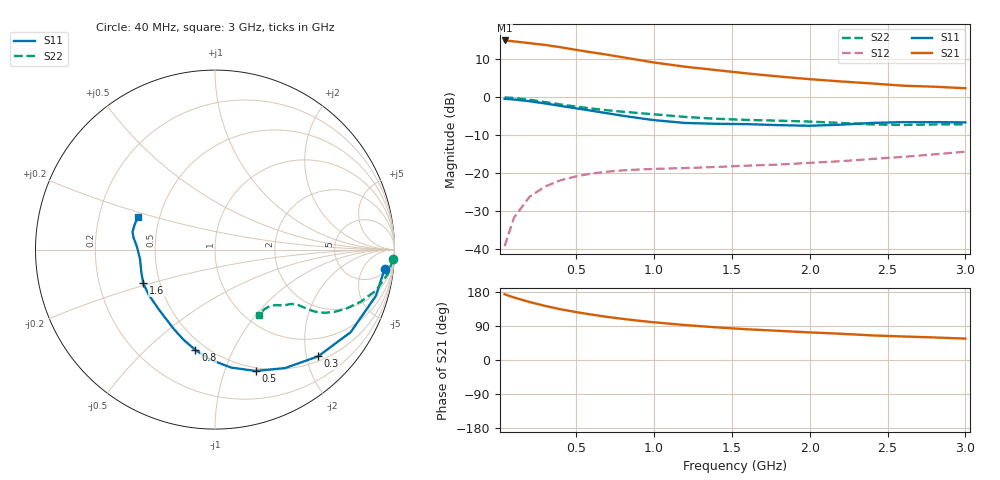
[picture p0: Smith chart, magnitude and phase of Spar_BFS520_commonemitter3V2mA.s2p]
! Filename:  BFS520A.S2P  Version:  4.0
! NXP part #: BFS520  Date: Jun 1994
! Bias condition: Vce=3V, Ic=2mA
#  MHz  S  MA  R  50
! Freq  S11  S21  S12  S22  !GUM [dB]
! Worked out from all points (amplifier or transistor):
!   21 points, 40 MHz to 3 GHz, reference 50 ohm
!   highest |S21| = 14.9 dB at 40 MHz (marker M1)
!   |S21| within 3 dB of that: start of sweep to 580.8 MHz
!   unconditionally stable (mu >= 1): 1.322 GHz to end of sweep
!   at 300 MHz: K = 0.28, MSG = 18.6 dB, |S12| = -23.5 dB
!   at 1 GHz: K = 0.78, MSG = 14.0 dB, |S12| = -18.9 dB
!   at 3 GHz: K = 1.19, MAG = 5.7 dB, |S12| = -14.3 dB
!   S11 on the Smith chart (normalised r, x): 40 MHz: 7, -15; 300 MHz: 0.59, -2.22; 500 MHz: 0.47, -1.28; 800 MHz: 0.44, -0.73; 1.6 GHz: 0.40, -0.19; 3 GHz: 0.38, +0.18
40  0.951 -6.5  5.567 173.5  0.011 85.2  0.992 -3.1
100  0.933 -16.0  5.416 165.0  0.026 79.0  0.976 -7.6
200  0.885 -31.3  5.128 153.0  0.049 69.6  0.925 -14.3
300  0.827 -46.0  4.862 142.8  0.067 62.0  0.862 -19.7
400  0.767 -59.4  4.532 133.8  0.081 56.2  0.803 -24.1
500  0.713 -71.5  4.186 126.4  0.091 51.9  0.751 -27.5
600  0.663 -82.3  3.885 119.8  0.099 48.9  0.708 -29.8
700  0.614 -92.3  3.615 113.7  0.105 47.1  0.673 -31.3
800  0.57 -101.0  3.342 108.5  0.109 45.9  0.644 -32.1
900  0.532 -109.2  3.088 103.7  0.112 44.9  0.619 -32.6
1000  0.499 -117.3  2.857 99.5  0.114 44.7  0.595 -33.0
1200  0.458 -132.8  2.514 92.2  0.117 45.2  0.55 -33.8
1400  0.447 -145.5  2.27 86.2  0.121 47.0  0.52 -35.6
1600  0.442 -154.8  2.05 81.0  0.126 49.3  0.502 -37.9
1800  0.429 -163.2  1.871 77.0  0.13 52.8  0.491 -39.4
2000  0.421 -172.9  1.725 72.8  0.137 56.2  0.478 -40.5
2200  0.435 178.0  1.61 69.3  0.144 59.9  0.458 -42.4
2400  0.459 171.6  1.514 64.9  0.154 62.9  0.438 -46.1
2600  0.47 167.8  1.416 62.1  0.164 65.4  0.431 -50.9
2800  0.469 163.3  1.373 59.5  0.177 68.6  0.438 -54.3
3000  0.467 156.9  1.311 56.5  0.192 70.8  0.44 -56.2
